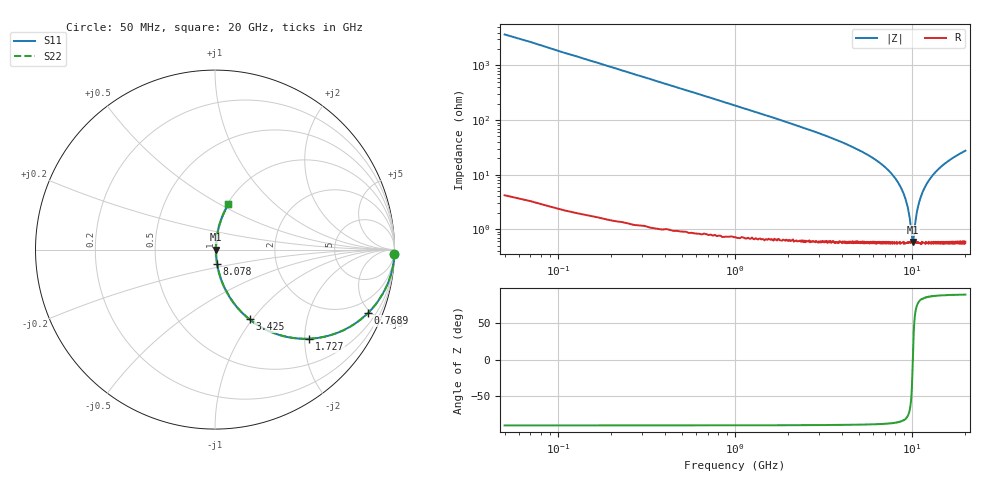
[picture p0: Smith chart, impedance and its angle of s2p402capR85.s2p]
! AVX Thin Film Operation		Date: September 2011
! Description: Accu-P® Series, Thin Film, SMD, RF Capacitor
! Part Number: 04021JR85ZBW/STR
! 50 MHz  -  20 GHz
! Serial Measurements
# MHZ S MA R 50
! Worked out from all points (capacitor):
!   1000 points, 50 MHz to 20 GHz, reference 50 ohm
!   read as one part in series: C = 851 fF near 149.8 MHz
!   lowest |Z| = 583 mohm at 10.09 GHz (marker M1)
!   series resonance near 10.1 GHz, so ESL is about 290 pH
!   S11 on the Smith chart (normalised r, x): 50 MHz: -0, -75; 768.9 MHz: 1.02, -4.84; 1.727 GHz: 1.01, -2.11; 3.425 GHz: 1.01, -0.97; 8.078 GHz: 1.01, -0.17; 20 GHz: 1.01, +0.55
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50  1 -1.5  0.027 88.4  0.027 88.4  1 -1.5
209.76  0.994 -6.4  0.111 83.5  0.111 83.5  0.994 -6.4
309.61  0.986 -9.4  0.163 80.5  0.163 80.5  0.986 -9.4
509.309  0.964 -15.2  0.263 74.6  0.263 74.6  0.964 -15.2
768.919  0.923 -22.4  0.381 67.4  0.381 67.4  0.923 -22.4
1727.477  0.723 -43.4  0.687 46.3  0.687 46.3  0.723 -43.4
3384.985  0.439 -63.3  0.893 26.0  0.893 26.0  0.439 -63.3
3424.925  0.433 -63.6  0.896 25.7  0.896 25.7  0.433 -63.6
6700  0.154 -79.1  0.983 8.8  0.983 8.8  0.154 -79.1
8077.928  0.083 -81.4  0.991 4.7  0.991 4.7  0.083 -81.4
8816.817  0.05 -80.8  0.993 2.9  0.993 2.9  0.05 -80.8
9356.006  0.029 -77.1  0.994 1.6  0.994 1.6  0.029 -77.1
9675.526  0.017 -69.5  0.994 0.9  0.994 0.9  0.017 -69.5
10034.99  0.006012 -21.5  0.994 0.1  0.994 0.1  0.006012 -21.5
10094.9  0.005588 -0.2  0.994 0.0  0.994 0.0  0.005588 -0.2
10194.75  0.006653 32.7  0.994 -0.2  0.994 -0.2  0.006653 32.7
10614.11  0.019 72.1  0.994 -1.1  0.994 -1.1  0.019 72.1
11153.3  0.037 79.3  0.994 -2.1  0.994 -2.1  0.037 79.3
12051.95  0.066 81.4  0.992 -3.8  0.992 -3.8  0.066 81.4
13350  0.104 81.0  0.989 -6.0  0.989 -6.0  0.104 81.0
16684.99  0.19 77.4  0.976 -10.9  0.976 -10.9  0.19 77.4
20000  0.263 73.6  0.959 -15.2  0.959 -15.2  0.263 73.6
